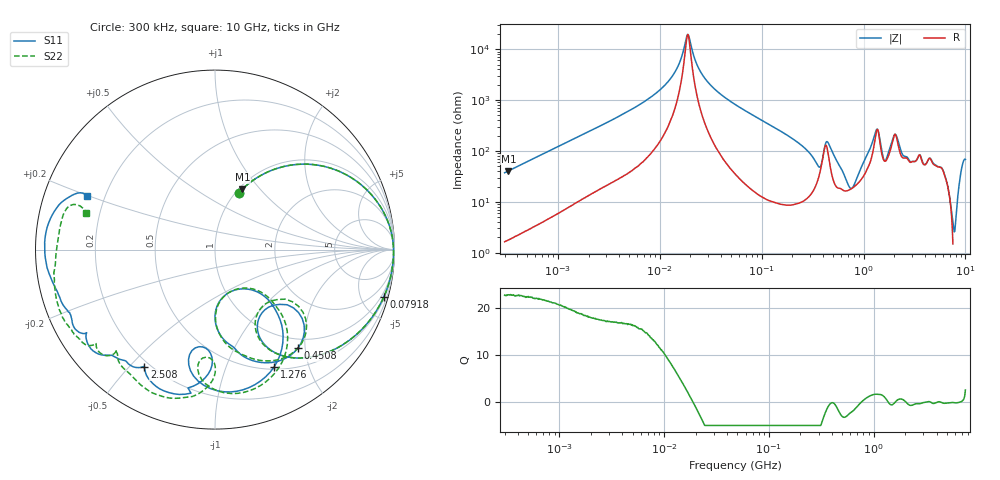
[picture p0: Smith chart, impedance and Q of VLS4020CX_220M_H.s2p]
! S-Parameter Data Generated by TDK Corporation
! Copyright(C) 2024 TDK Corporation.
! All Rights Reserved.
! TDK P/N: VLS4020CX-220M-H (SMD / SMT Inductor (Coil))
! Property: L=22uH at 1MHz
! Size(LxWxT): 4x4x2mm
! Model Type: s2p (Touchstone File Format Version 1.0)
! Frequency: DC=Yes Start=0.3MHz Stop=10000MHz 802points Log-sweep
! Model Generated on May 28, 2024
! Terms and conditions regarding TDK Simulation Models:
! 1)This simulation model is being provided solely for informational
!  purposes. Please refer to the specifications of the products in
!  terms of detailed characteristics of such products.
! 2)In no event shall TDK Corporation of any of its subsidiaries be
!  liable for any loss or damage arising, directly or indirectly,
!  from any information contained in this simulation model, including,
!  but not limited to loss or damages arising from any inaccuracies,
!  omissions or errors in connection with such information.
! 3)Any and all copyrights on this simulation model are owned by
!  TDK Corporation.  Duplication or redistribution of this simulation
!  model without prior written permission from TDK Corporation
!  is prohibited.
! 4)This simulation model is subject to any modification or change
!  without any prior notice.
! 5)Neither TDK Corporation nor any of its subsidiaries shall make any
!  warranty, express or implied, including but not limited to the
!  correctness, implied warranties of merchantability and fitness for
!  a particular purpose with respect to this simulation models.
! 6)The use of this simulation model shall be deemed to have consented
!  to the terms and conditions hereof.
! Port Assignments:
!  1 ---@@@--- 2
! Applicable Conditions:
!  Temperature = 25 degC
!  DC Bias Current = 0 A
!  Small Signal Operation
# Hz S MA R 50
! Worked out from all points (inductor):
!   801 points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, 300 kHz to 10 GHz, reference 50 ohm
!   read as one part in series: L = 19.7 uH near 318.3 kHz
!   highest Q = 22.8 at 327.5 kHz (marker M1), where L = 19.7 uH
!   self-resonance near 18.77 MHz
!   S11 on the Smith chart (normalised r, x): 300 kHz: 1.03, +0.74; 79.18 MHz: 0.63, -7.23; 450.8 MHz: 0.82, -1.86; 1.276 GHz: 0.53, -1.49; 2.508 GHz: 0.18, -0.55; 10 GHz: 0.13, +0.20
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300000  0.3432 67.3  0.9241 -20.2  0.9241 -20.2  0.3434 67.3
327506  0.3698 65.7  0.9129 -21.8  0.9131 -21.8  0.3699 65.7
1713600  0.8803 25.2  0.4289 -61.6  0.429 -61.7  0.8804 25.2
9671944  0.9916 3.2  0.06675 -81.5  0.06677 -81.5  0.9916 3.2
1.421446e7  0.9942 0.6  0.02719 -77.9  0.02719 -78.0  0.9943 0.6
1.899897e7  0.9949 -1.3  0.005124 6.3  0.005127 6.3  0.995 -1.3
2.819857e7  0.9943 -4.0  0.0389 78.9  0.03892 78.9  0.9944 -4.0
5.477226e7  0.9877 -10.4  0.1196 77.2  0.1196 77.2  0.9877 -10.3
7.918232e7  0.9768 -15.6  0.184 72.5  0.184 72.5  0.9768 -15.6
3.126428e8  0.653 -60.4  0.6613 20.4  0.6615 20.4  0.6496 -60.7
3.910695e8  0.4491 -43.6  0.6 -11.1  0.6001 -11.1  0.4237 -42.4
4.508285e8  0.7174 -49.9  0.4135 10.0  0.4135 10.0  0.7105 -47.1
7.318083e8  0.4056 -89.7  0.7671 -21.1  0.7672 -21.1  0.4091 -89.3
1.001841e9  0.3028 -47.8  0.6982 -62.1  0.6983 -62.1  0.2973 -47.0
1.276148e9  0.7318 -63.2  0.2951 -94.8  0.2952 -94.8  0.7295 -59.2
1.547353e9  0.6875 -101.5  0.3644 -49.5  0.3649 -49.5  0.7264 -95.9
1.767019e9  0.5788 -92.4  0.3674 -89.9  0.3677 -90.0  0.6484 -89.9
2.051294e9  0.8226 -101.7  0.157 -83.8  0.1571 -83.9  0.8493 -103.1
2.507534e9  0.7631 -121.1  0.2376 -73.7  0.2375 -73.9  0.8417 -123.5
5.607117e9  0.8876 -156.9  0.09889 -119.2  0.09888 -119.2  0.919 -151.6
7.316673e9  0.9434 -175.4  0.07696 -126.5  0.07686 -126.4  0.8993 -173.2
1e10  0.771 157.3  0.05251 -126.5  0.05262 -126.6  0.7454 163.9
